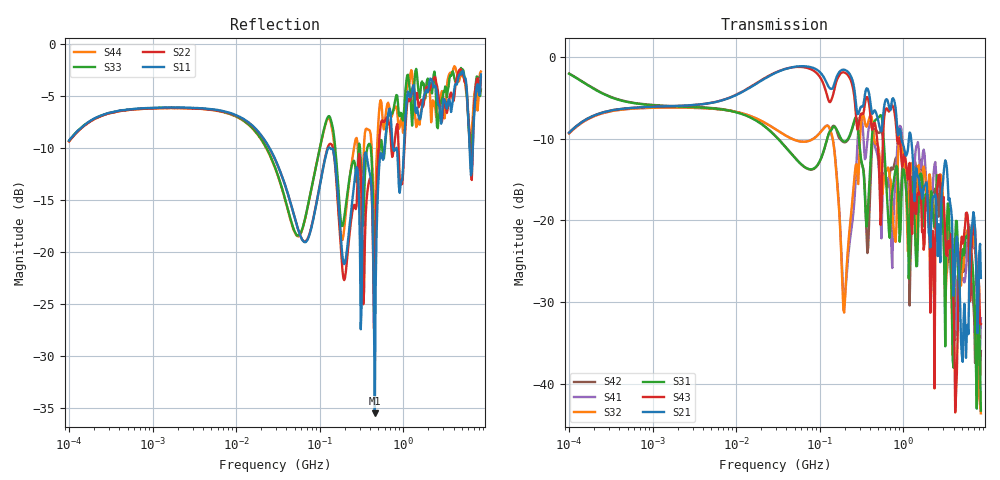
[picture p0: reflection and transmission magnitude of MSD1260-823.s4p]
# MHz S MA R 50
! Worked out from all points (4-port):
!   498 points, 100 kHz to 8.5 GHz, reference 50 ohm
!   strongest paths, dB at 100 kHz, 1.698 MHz, 29.49 MHz, 500.7 MHz, 8.5 GHz:
!     S21: -9.3, -6.0, -2.0, -7.8, -27.0
!     S43: -9.3, -6.0, -1.9, -11.5, -32.7
!     S31: -2.1, -6.0, -9.7, -7.5, -43.3
!     S32: -9.3, -6.2, -8.8, -10.9, -43.6
!     S41: -9.4, -6.2, -8.8, -12.6, -32.0
!     S42: -2.0, -6.0, -9.7, -9.3, -36.0
!   lowest |S11| = -35.5 dB at 457 MHz (marker M1), VSWR 1.03, Z = 51.5 + j0.813 ohm
!   |S11| at or under -10 dB: 132.9 MHz to 596.1 MHz (463.2 MHz wide, 127 % of centre); 829.1 MHz to 1.018 GHz (189.2 MHz wide, 20.5 % of centre); 6.237 GHz to 6.798 GHz (561.6 MHz wide, 8.62 % of centre)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
0.1  0.3431 44.7  0.3445 45.5  0.7896 -18.1  0.3408 -135.1
     0.3445 45.5  0.3407 44.9  0.3409 -135.1  0.791 -18.1
     0.7896 -18.1  0.3409 -135.1  0.3439 44.8  0.3438 45.4
     0.3408 -135.1  0.791 -18.1  0.3438 45.4  0.3406 44.9
124.3153  0.3111 -6.8  0.6742 -31.7  0.3228 157.6  0.3803 5.5
          0.6742 -31.7  0.3173 -8.3  0.3798 6.3  0.322 156.4
          0.3228 157.6  0.3798 6.3  0.4437 -6.0  0.5653 -38.2
          0.3803 5.5  0.322 156.4  0.5653 -38.2  0.4368 -7.5
196.287  0.08767 -24.4  0.8347 -41.3  0.3035 51.3  0.03222 -10.6
         0.8347 -41.3  0.07347 -24.6  0.02732 4.4  0.3005 47.8
         0.3035 51.3  0.02732 4.4  0.1463 -8.5  0.8039 -46.5
         0.03222 -10.6  0.3005 47.8  0.8039 -46.5  0.1291 1.7
456.9518  0.01685 27.9  0.4718 -80.9  0.4074 -8.6  0.2849 -60.0
          0.4718 -80.9  0.07697 37.1  0.3006 -58.6  0.3625 -16.0
          0.4074 -8.6  0.3006 -58.6  0.09804 -24.6  0.3944 -97.1
          0.2849 -60.0  0.3625 -16.0  0.3944 -97.1  0.1468 4.6
2312.454  0.6185 174.8  0.1399 94.1  0.09973 119.6  0.1956 126.5
          0.1399 94.1  0.6799 179.2  0.1145 108.2  0.157 112.1
          0.09973 119.6  0.1145 108.2  0.7113 174.0  0.06642 81.9
          0.1956 126.5  0.157 112.1  0.06642 81.9  0.5314 173.5
3735.583  0.4713 4.1  0.1171 -160.3  0.04331 -65.9  0.06235 -38.5
          0.1171 -160.3  0.5843 -7.3  0.04491 -56.8  0.05807 -57.0
          0.04331 -65.9  0.04491 -56.8  0.7024 -2.2  0.08253 -172.5
          0.06235 -38.5  0.05807 -57.0  0.08253 -172.5  0.7224 -1.0
8500  0.7134 -32.3  0.0445 -135.1  0.006868 -59.5  0.02523 -73.3
      0.0445 -135.1  0.6898 -40.5  0.006612 -85.2  0.01589 -80.2
      0.006868 -59.5  0.006612 -85.2  0.6044 -36.3  0.02324 -125.3
      0.02523 -73.3  0.01589 -80.2  0.02324 -125.3  0.737 -46.0
